(* Logix 5000 DataType export TeNod4TCYCIN; software revision 28.00 *)

TYPE TeNod4TCYCIN :
STRUCT
   eNodCounter : DINT;
   MeasureStatus : TeNod4TStatus;
   Gross : DINT;
   Tare : DINT;
   Net : DINT;
   ADCPoints : DINT;
   CommandEcho : INT;
   Response : INT;
END_STRUCT
END_TYPE

TYPE TeNod4TStatus :
STRUCT
   Reserved : INT;
   b00Reserved : BOOL;
   b01Reserved : BOOL;
   b02ErrorCode0 : BOOL;
   b03ErrorCode1 : BOOL;
   b04NoMotion : BOOL;
   b05ZeroWeight : BOOL;
   b06EEPROMFailure : BOOL;
   b07Reserved : BOOL;
   b08Input1ON : BOOL;
   b09Input2ON : BOOL;
   b10Output1ON : BOOL;
   b11Output2ON : BOOL;
   b12Output3ON : BOOL;
   b13Output4ON : BOOL;
   b14TareActive : BOOL;
   b15Reservd : BOOL;
END_STRUCT
END_TYPE
